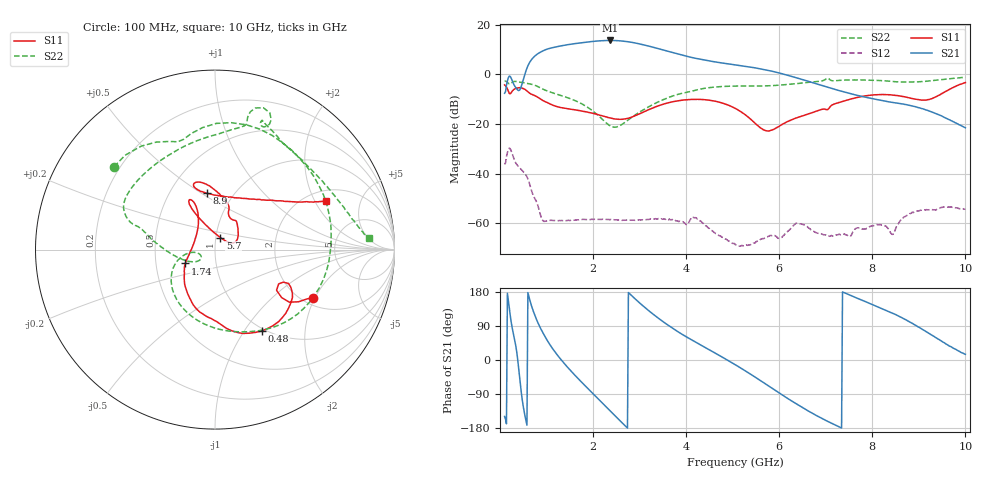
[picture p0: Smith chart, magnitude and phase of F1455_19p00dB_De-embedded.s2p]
! Integrated Device Technology
! Corporate Headquarters
! 6024 Silver Creek Valley Road
! San Jose, CA 95138  USA
! Phone:  1-408-284-8200
! Toll Free:  1-800-223-1366
! Webpage:  http://www.idt.com/
! Timing and RF Division
! 515 Groton Road, Suite 102
! Westford, MA 01886-6024
! Device:  F1455
! Description: 6-bit 0.5 dB Transmit Variable Gain Amplifier
! Frequency:  1400.0 -  2300.00 MHz
! Package:  6x6 mm Thin QFN Plastic Package: 28 pin
! State:  38
! Atten State:  19.0 dB
! Voltage:  +5.00 Volts
! Current:  217.630 mA
! Data:  The device was measured on a the F1455 evaluation board which has
!  individual transmission lines to the RF pins.  Data was collected
!  using a calibrated network analyzer.  The evaluation board was
!  de-embedded using a TRL calibration technique.
!  The reference plane is the edge of the package pin.
!  Pin  1 = CSb
!  Pin  2 = DATA
!  Pin  3 = CLK
!  Pin  4 = RSET
!  Pin  5 = GND
!  Pin  6 = RFIN  = Port 1
!  Pin  7 = GND
!  Pin  8 = NC
!  Pin  9 = NC
!  Pin 10 = NC
!  Pin 11 = NC
!  Pin 12 = NC
!  Pin 13 = NC
!  Pin 14 = /STBY
!  Pin 15 = GND
!  Pin 16 = RFOUT  = Port 2
!  Pin 17 = GND
!  Pin 18 = NC
!  Pin 19 = NC
!  Pin 20 = NC
!  Pin 21 = GND
!  Pin 22 = NC
!  Pin 23 = GND
!  Pin 24 = NC
!  Pin 25 = NC
!  Pin 26 = NC
!  Pin 27 = GND
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# GHz S dB R 50
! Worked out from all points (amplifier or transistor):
!   496 points, 100 MHz to 10 GHz, reference 50 ohm
!   highest |S21| = 13.6 dB at 2.36 GHz (marker M1)
!   |S21| within 3 dB of that: 1.107 GHz to 3.343 GHz (2.236 GHz wide, 101 % of centre)
!   unconditionally stable (mu >= 1): start of sweep to end of sweep
!   at 1.74 GHz: K = 87.98, MAG = 13.1 dB, |S12| = -58.5 dB
!   at 5.06 GHz: K = 565.60, MAG = 5.7 dB, |S12| = -68.7 dB
!   at 10 GHz: K = 430.36, MAG = -13.0 dB, |S12| = -54.3 dB
!   S11 on the Smith chart (normalised r, x): 100 MHz: 2.26, -1.92; 480 MHz: 0.97, -1.21; 1.74 GHz: 0.71, -0.11; 5.7 GHz: 1.05, +0.14; 8.9 GHz: 0.75, +0.53; 10 GHz: 2.47, +2.49
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0.1  -4.33 -26.2  -7.67 -148.9  -36.33 46.8  -2.76 140.7
0.26  -6.91 -24.7  -2.47 86.7  -31.89 -76.7  -3.30 95.7
0.38  -5.51 -41.8  -6.35 2.7  -36.80 -116.9  -3.05 57.8
0.48  -5.63 -60.1  -3.57 -105.8  -38.83 -148.3  -3.35 31.6
0.68  -8.10 -90.7  5.92 142.1  -47.00 140.5  -4.06 -15.3
0.82  -9.37 -109.0  8.32 97.1  -53.22 114.8  -5.03 -46.6
0.96  -10.96 -123.3  9.71 63.6  -59.27 125.3  -6.34 -71.9
1.32  -13.48 -143.8  11.44 -0.1  -58.90 96.7  -8.64 -119.6
1.74  -14.74 -155.1  12.65 -56.7  -58.46 63.6  -11.74 -155.2
1.76  -14.81 -155.5  12.70 -59.3  -58.52 62.3  -11.94 -156.6
2.06  -16.01 -164.1  13.31 -96.3  -58.48 45.5  -15.80 -171.4
2.36  -17.60 179.7  13.59 -133.3  -58.60 32.6  -20.70 -165.6
2.78  -17.63 141.9  12.99 175.6  -58.76 20.2  -18.11 -147.5
3.08  -15.29 122.5  11.85 142.1  -58.67 13.2  -14.34 -163.7
3.4  -12.76 114.7  10.30 110.6  -58.16 2.5  -11.19 -179.6
4.08  -10.18 116.1  6.90 55.8  -58.88 -10.0  -7.01 163.3
5.06  -13.80 117.3  3.75 -12.7  -68.71 -33.7  -4.78 148.0
5.7  -22.66 65.9  1.78 -62.7  -65.87 -7.7  -4.71 121.9
6.7  -15.59 39.6  -3.29 -139.8  -62.81 -128.2  -3.15 78.4
8.36  -8.27 107.7  -11.15 127.2  -62.84 111.4  -2.79 62.3
8.9  -9.98 98.3  -13.00 93.6  -55.43 125.0  -3.14 40.7
10  -3.38 23.8  -21.58 15.0  -54.33 45.9  -1.28 4.5
